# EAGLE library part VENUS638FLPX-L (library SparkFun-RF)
Venus638FLPX-L GPS Receiver Venus638FLPx is a high performance, low cost, single chip GPS receiver targeting mobile consumer and cellular handset applications. It offers very low power consumption, high sensitivity, and best in class signal acquisition and time-to-first-fix performance. Venus638FLPx contains all the necessary components of a complete GPS receiver, includes 1.2dB cascaded system NF RF front-end, GPS baseband signal processor, 0.5ppm TCXO, 32.768kHz RTC crystal, RTC LDO regulator, and passive components. It requires very low external component count and takes up only 100mm2 PCB footprint. Dedicated massive-correlator signal parameter search engine within the baseband enables rapid search of all the available satellites and acquisition of very weak signal. An advanced track engine allows weak signal tracking and positioning in harsh environments such as urban canyons and under deep foliage. The self-contained architecture keeps GPS processing off the host and allows integration into applications with very little resource. FEATURES 20Hz update rate -148dBm cold start sensitivity -165dBm tracking sensitivity 29 second cold start TTFF 3.5 second TTFF with AGPS 1 second hot start 2.5m accuracy Multipath detection and suppression Jamming detection and mitigation SBAS (WAAS / EGNOS) support 7-day extended ephemeris AGPS 67mW full power navigation Works directly with active or passive antenna Internal flash for optional 75K point data logging Supports external SPI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
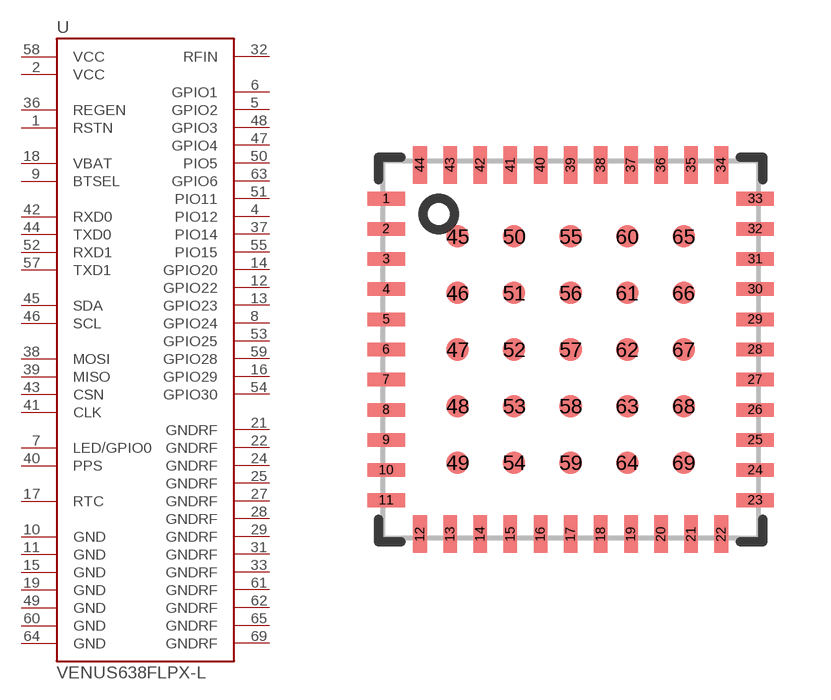
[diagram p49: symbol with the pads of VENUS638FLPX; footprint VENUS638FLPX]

Designator prefix U

## VENUS638FLPX-L  [VENUS638FLPX]
1  RSTN
2  VCC
4  PIO12
5  GPIO2
6  GPIO1
7  LED/GPIO0
8  GPIO24
9  BTSEL
10  GND
11  GND
12  GPIO22
13  GPIO23
14  GPIO20
15  GND
16  GPIO29
17  RTC
18  VBAT
19  GND
21  GNDRF
22  GNDRF
24  GNDRF
25  GNDRF
27  GNDRF
28  GNDRF
29  GNDRF
31  GNDRF
32  RFIN
33  GNDRF
36  REGEN
37  PIO14
38  MOSI
39  MISO
40  PPS
41  CLK
42  RXD0
43  CSN
44  TXD0
45  SDA
46  SCL
47  GPIO4
48  GPIO3
49  GND
50  PIO5
51  PIO11
52  RXD1
53  GPIO25
54  GPIO30
55  PIO15
57  TXD1
58  VCC
59  GPIO28
60  GND
61  GNDRF
62  GNDRF
63  GPIO6
64  GND
65  GNDRF
69  GNDRF

## Footprint VENUS638FLPX (pad centres in mm)
smd 1 x 0.36: 1 -4.9,4; 2 -4.9,3.2; 3 -4.9,2.4; 4 -4.9,1.6; 5 -4.9,0.8; 6 -4.9,0; 7 -4.9,-0.8; 8 -4.9,-1.6; 9 -4.9,-2.4; 10 -4.9,-3.2; 11 -4.9,-4; 23 4.9,-4; 24 4.9,-3.2; 25 4.9,-2.4; 26 4.9,-1.6; 27 4.9,-0.8; 28 4.9,0; 29 4.9,0.8; 30 4.9,1.6; 31 4.9,2.4; 32 4.9,3.2; 33 4.9,4
smd 0.36 x 1: 12 -4,-4.9; 13 -3.2,-4.9; 14 -2.4,-4.9; 15 -1.6,-4.9; 16 -0.8,-4.9; 17 0,-4.9; 18 0.8,-4.9; 19 1.6,-4.9; 20 2.4,-4.9; 21 3.2,-4.9; 22 4,-4.9; 34 4,4.9; 35 3.2,4.9; 36 2.4,4.9; 37 1.6,4.9; 38 0.8,4.9; 39 0,4.9; 40 -0.8,4.9; 41 -1.6,4.9; 42 -2.4,4.9; 43 -3.2,4.9; 44 -4,4.9
smd 0.6 x 0.6: 45 -3,3; 46 -3,1.5; 47 -3,0; 48 -3,-1.5; 49 -3,-3; 50 -1.5,3; 51 -1.5,1.5; 52 -1.5,0; 53 -1.5,-1.5; 54 -1.5,-3; 55 0,3; 56 0,1.5; 57 0,0; 58 0,-1.5; 59 0,-3; 60 1.5,3; 61 1.5,1.5; 62 1.5,0; 63 1.5,-1.5; 64 1.5,-3; 65 3,3; 66 3,1.5; 67 3,0; 68 3,-1.5; 69 3,-3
